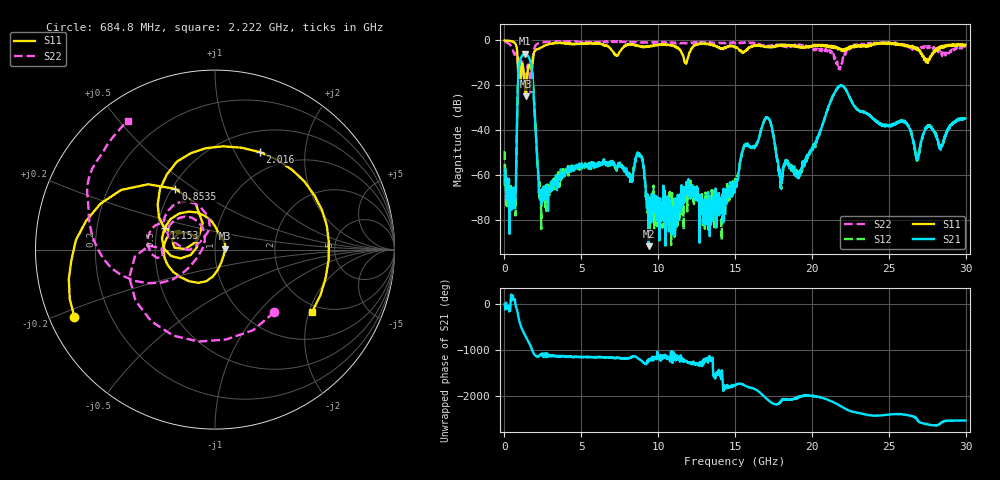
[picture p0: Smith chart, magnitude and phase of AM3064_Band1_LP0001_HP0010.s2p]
# Hz S DB R 50.0
!freq dBS11 angS11 dBS21 angS21 dBS12 angS12 dBS22 angS22
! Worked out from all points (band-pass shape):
!   1600 points, 10 MHz to 29.98 GHz, reference 50 ohm
!   highest |S21| = -5.87 dB at 1.341 GHz (marker M1); lowest = -91.9 dB at 9.382 GHz (marker M2)
!   |S21| within 3 dB of the highest: 1.013 GHz to 1.676 GHz (662.7 MHz wide, 49.3 % of centre)
!   lowest |S11| = -25.0 dB at 1.397 GHz (marker M3), VSWR 1.12, Z = 56 + j0.544 ohm
!   |S11| at or under -10 dB: 865.8 MHz to 1.83 GHz (963.7 MHz wide, 71.5 % of centre); 11.74 GHz to 11.84 GHz (101.7 MHz wide, 0.862 % of centre); 27.52314 GHz to 27.54176 GHz (18.61 MHz wide, 0.0676 % of centre)
!   |S22| runs from -23.2 to -0.2 dB; largest |S21 - S12| = 0.0058
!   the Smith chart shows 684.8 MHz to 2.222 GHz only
!   S11 on the Smith chart (normalised r, x): 684.8 MHz: 0.07, -0.23; 853.5 MHz: 0.52, +0.42; 1.153 GHz: 0.55, +0.15; 2.016 GHz: 0.75, +1.26; 2.222 GHz: 1.76, -2.09
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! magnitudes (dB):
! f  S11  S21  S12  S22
! 10 MHz  0.0  -60.2  -49.5  -0.2
! 253.7 MHz  -0.2  -74.1  -67.5  -1.3
! 684.8 MHz  -1.2  -71.0  -70.8  -6.4
! 853.5 MHz  -7.9  -25.2  -25.1  -8.7
! 1.153 GHz  -10.3  -7.0  -6.9  -9.7
! 1.341 GHz  -22.5  -5.9  -5.8  -19.7
! 1.397 GHz  -25.0  -6.0  -6.0  -16.1
! 1.734 GHz  -12.8  -10.4  -10.4  -20.2
! 2.016 GHz  -4.5  -38.5  -38.4  -2.4
! 2.222 GHz  -3.8  -62.2  -62.9  -1.3
! 5.015 GHz  -1.3  -55.9  -57.9  -0.7
! 8.801 GHz  -2.6  -51.7  -50.9  -0.9
! 9.382 GHz  -2.7  -91.9  -77.3  -0.9
! 10 GHz  -2.0  -72.8  -75.8  -0.9
! 15 GHz  -3.0  -64.3  -61.9  -1.3
! 17.05 GHz  -2.9  -34.5  -34.3  -2.6
! 17.97 GHz  -2.4  -65.9  -62.4  -2.1
! 19.99 GHz  -2.8  -48.4  -48.4  -3.3
! 21.83 GHz  -3.8  -20.4  -20.2  -13.0
! 25 GHz  -1.0  -38.0  -38.4  -1.1
! 26.87 GHz  -4.1  -53.6  -53.3  -3.2
! 29.98 GHz  -1.9  -34.9  -35.0  -3.2
